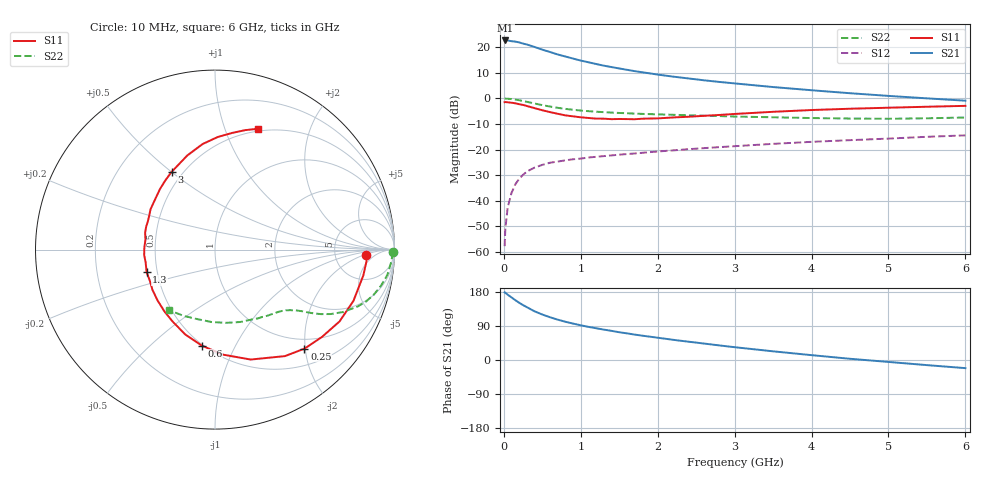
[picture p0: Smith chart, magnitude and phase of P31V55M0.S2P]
! SIEMENS Small Signal Semiconductors
! BFP181
! Si NPN RF Bipolar Junction Transistor in SOT143
! VCE = 1.5 V  IC = 5 mA
! Common Emitter S-Parameters:  March  1996
# GHz  S  MA  R  50
!  f  S11  S21  S12  S22
! GHz  MAG  ANG  MAG  ANG  MAG  ANG  MAG  ANG
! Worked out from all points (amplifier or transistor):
!   36 points, 10 MHz to 6 GHz, reference 50 ohm
!   highest |S21| = 22.6 dB at 20 MHz (marker M1)
!   |S21| within 3 dB of that: start of sweep to 443.7 MHz
!   unconditionally stable (mu >= 1): 1.534 GHz to end of sweep
!   at 250 MHz: K = 0.24, MSG = 25.6 dB, |S12| = -29.8 dB
!   at 1.4 GHz: K = 0.96, MSG = 17.2 dB, |S12| = -22.3 dB
!   at 6 GHz: K = 1.07, MAG = 5.2 dB, |S12| = -14.4 dB
!   S11 on the Smith chart (normalised r, x): 10 MHz: 11, -2; 250 MHz: 0.80, -1.99; 600 MHz: 0.49, -0.74; 1.3 GHz: 0.44, -0.13; 3 GHz: 0.44, +0.50; 6 GHz: 0.47, +1.30
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0.01  0.8416 -2.1  13.46 178.6  0.0013 92.1  0.9892 -0.8
0.02  0.8468 -4.3  13.52 177.4  0.0029 88.8  0.9892 -1.7
0.05  0.8386 -10.0  13.52 172.4  0.0074 87.1  0.9835 -4.3
0.15  0.801 -30.0  12.84 157.8  0.0211 74.6  0.9464 -12.3
0.2  0.7695 -39.2  12.38 151.0  0.0269 69.0  0.9192 -15.9
0.25  0.7437 -47.9  11.74 144.8  0.0322 64.8  0.8895 -19.0
0.3  0.71 -56.7  11.26 139.3  0.0373 61.5  0.8564 -21.7
0.4  0.6441 -72.0  10.09 128.4  0.0446 55.6  0.7935 -26.0
0.5  0.5867 -85.7  8.94 120.0  0.0503 50.2  0.7383 -29.1
0.6  0.5398 -97.9  8.05 112.8  0.0554 47.4  0.6921 -31.3
0.7  0.5007 -109.4  7.202 106.5  0.0583 45.0  0.6541 -32.9
0.8  0.4659 -120.2  6.569 100.9  0.0617 43.1  0.6239 -34.1
0.9  0.4457 -129.0  5.987 96.1  0.0647 41.7  0.5984 -35.1
1.1  0.4144 -147.2  5.069 87.4  0.07 40.1  0.5625 -37.0
1.3  0.4012 -161.9  4.352 80.2  0.0746 38.9  0.5381 -38.8
1.7  0.3914 171.9  3.407 67.1  0.0839 38.0  0.5044 -42.8
2.2  0.424 147.7  2.66 53.3  0.0965 36.6  0.4777 -49.1
3  0.4962 119.1  1.961 33.8  0.1165 33.3  0.4417 -61.4
3.5  0.5467 106.4  1.664 22.9  0.1294 30.6  0.4273 -70.7
4.5  0.6276 88.6  1.261 3.2  0.1528 24.4  0.4041 -92.5
5.5  0.6866 75.8  1.001 -13.5  0.1778 18.6  0.4086 -115.4
6  0.7142 70.5  0.901 -21.5  0.1895 14.9  0.4233 -127.0
